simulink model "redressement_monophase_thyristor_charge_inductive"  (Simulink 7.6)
settings: Solver=FixedStepDiscrete  StartTime=0.0  StopTime=N  RelTol=1e-3
InitFcn:
  | clc
  | clear all
  | close all
  | Ts=1e-5;
  | N=0.035;
StopFcn:
  | subplot 211
  | load iAK_vAK.mat
  | plot(x(1,:),x(2,:))
  | grid
  | title('Courant iAK - redressement monophasé, charge inductive à thyristor')
  | axis([0 N -1 100000])
  | 
  | subplot 212
  | plot(x(1,:),x(3,:))
  | xlabel('temps')
  | title('Tension vAK - redressement monophasé, charge inductive à thyristor')
  | grid
  | axis([0 N -150 100])
  | 
  | figure
  | load Ug_vs.mat
  | subplot 211
  | plot(y(1,:),y(2,:))
  | title('Tension de sortie vs - redressement monophasé, charge inductive à thyristor')
  | axis([0 N -100 120])
  | grid
  | 
  | subplot 212
  | plot(y(1,:),y(3,:))
  | grid
  | axis([0 N -0.2 1.2])
  | title('Tension de commande de la gâchette - redressement monophasé, charge inductive à thyristor')
  | xlabel('temps')
undefined symbols (not defined in the file or in its folder): arm, bridge, pulses
libraries: powerlib x10, powerlib_extras x1

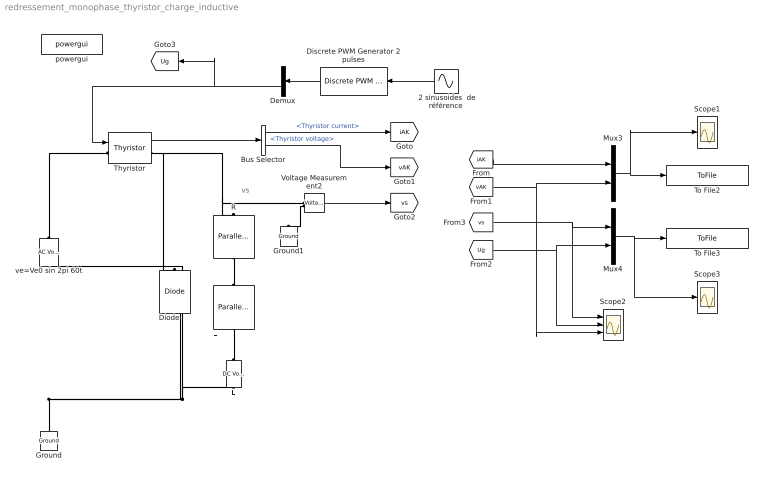
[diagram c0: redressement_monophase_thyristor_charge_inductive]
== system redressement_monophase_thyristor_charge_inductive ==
  note: vs
  " 2 sinusoides  de référence" : Sin  Frequency=2*pi*60  Phase=pi/3  SampleTime=Ts
  Bus Selector : BusSelector  OutputSignals=Thyristor current,Thyristor voltage
  Demux : Demux  Outputs=2
  Diode : powerlib/Power Electronics/Diode  DialogController=POWERSYS.PowerSysDialog  SystemSampleTime=-1  Ron=0.001  Lon=0  Vf=0.8  IC=0  UseSnubber=off  Rs=500  Cs=250e-9  Measurements=on
  Discrete PWM Generator 2 pulses : powerlib_extras/Discrete  Control Blocks/Discrete PWM Generator  DialogController=POWERSYS.PowerSysDialog  SystemSampleTime=-1  GeneratorMode="1-arm  bridge (2 pulses)"  Fc=1080  Ts=Ts  Internal=off  mIndex=0.8  Freq=60  Phase=0
  E : powerlib/Electrical Sources/DC Voltage Source  DialogController=POWERSYS.PowerSysDialog  SystemSampleTime=-1  Amplitude=80  Measurements=None
  Ground : powerlib/Elements/Ground  DialogController=POWERSYS.PowerSysDialog  PhysicalDomain=powersysdomain  SubClassName=unknown  LeftPortType=p1  RightPortType=p1  LConnTagsString=a
  Ground1 : powerlib/Elements/Ground  DialogController=POWERSYS.PowerSysDialog  PhysicalDomain=powersysdomain  SubClassName=unknown  LeftPortType=p1  RightPortType=p1  LConnTagsString=a
  L : powerlib/Elements/Parallel RLC Branch  DialogController=POWERSYS.PowerSysDialog  PhysicalDomain=powersysdomain  SubClassName=unknown  LeftPortType=p1  RightPortType=p1  LConnTagsString=a  RConnTagsString=__new0  BranchType=L  Resistance=1  Inductance=0.5  SetiL0=off  InitialCurrent=0  Capacitance=1e-6  Setx0=off  InitialVoltage=0  Measurements=None
  Mux3 : Mux  Inputs=2
  Mux4 : Mux  Inputs=2
  R : powerlib/Elements/Parallel RLC Branch  DialogController=POWERSYS.PowerSysDialog  PhysicalDomain=powersysdomain  SubClassName=unknown  LeftPortType=p1  RightPortType=p1  LConnTagsString=a  RConnTagsString=__new0  BranchType=R  Resistance=12  Inductance=1e-3  SetiL0=off  InitialCurrent=0  Capacitance=1e-6  Setx0=off  InitialVoltage=0  Measurements=None
  Scope1 : Scope
  Scope2 : Scope  NumInputPorts=3
  Scope3 : Scope
  Thyristor : powerlib/Power Electronics/Thyristor  DialogController=POWERSYS.PowerSysDialog  SystemSampleTime=-1  Ron=0.001  Lon=0  Vf=0.8  IC=0  Rs=500  Cs=250e-9  Measurements=on
  To File2 : ToFile  Filename=iAK_vAK  MatrixName=x
  To File3 : ToFile  Filename=Ug_vs  MatrixName=y
  Voltage Measurement2 : powerlib/Measurements/Voltage Measurement  DialogController=POWERSYS.PowerSysDialog  SystemSampleTime=-1  PhasorSimulation=off  OutputType=Complex  PSBequivalent=0
  powergui : powerlib/powergui  SystemSampleTime=-1  SimulationMode=Discrete  SampleTime=Ts  frequency=60  SPID=off  DisableSnubberDevices=off  DisableRonSwitches=off  DisableVfSwitches=off  SwTol=0  Interpol=off  frequencyindice=0  echomessages=off  HookPort=off  DisplayEquations=off  FunctionMessages=off  EnableUseOfTLC=off  x0status=blocks  RestoreLinks=warning  ResistiveCurrentMeasurement=off  Frange=[0:2:500]  Ylog=off  Xlog=on  ShowGrid=off  save=off  variable=ZData  ZoomFFT=on  StartTime=0.0  cycles=1  DisplayStyle=1  fundamental=60  FreqAxis=off  MaxFrequency=1000  frequencyindicesteady=60  RmsSteady=1  display=off  Ts=0  methode=off
  ve=Ve0 sin 2pi 60t : powerlib/Electrical Sources/AC Voltage Source  DialogController=POWERSYS.PowerSysDialog  SystemSampleTime=-1  Amplitude=100  Phase=0  Frequency=60  SampleTime=Ts  Measurements=None
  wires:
  Thyristor/1 -> Bus Selector/1
  Bus Selector/1 -> [iAK]  "<Thyristor current>"
  Bus Selector/2 -> [vAK]  "<Thyristor voltage>"
  Voltage Measurement2/1 -> [vs]
  [iAK] -> Mux3/1
  [vAK] -> Mux3/2, Scope2/3
  Mux3/1 -> To File2/1, Scope1/1
  Mux4/1 -> To File3/1, Scope3/1
  [Ug] -> Mux4/2, Scope2/2
  [vs] -> Mux4/1, Scope2/1
  " 2 sinusoides  de référence"/1 -> Discrete PWM Generator 2 pulses/1
  Discrete PWM Generator 2 pulses/1 -> Demux/1
  Demux/2 -> [Ug], Thyristor/1
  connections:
  Ground/LConn1 -- ve=Ve0 sin 2pi 60t/LConn1 -- E/LConn1 -- Diode/RConn1
  ve=Ve0 sin 2pi 60t/RConn1 -- Thyristor/LConn1
  Thyristor/RConn1 -- R/LConn1 -- Voltage Measurement2/LConn1 -- Diode/LConn1
  Voltage Measurement2/LConn2 -- Ground1/LConn1
  R/RConn1 -- L/LConn1
  L/RConn1 -- E/RConn1
